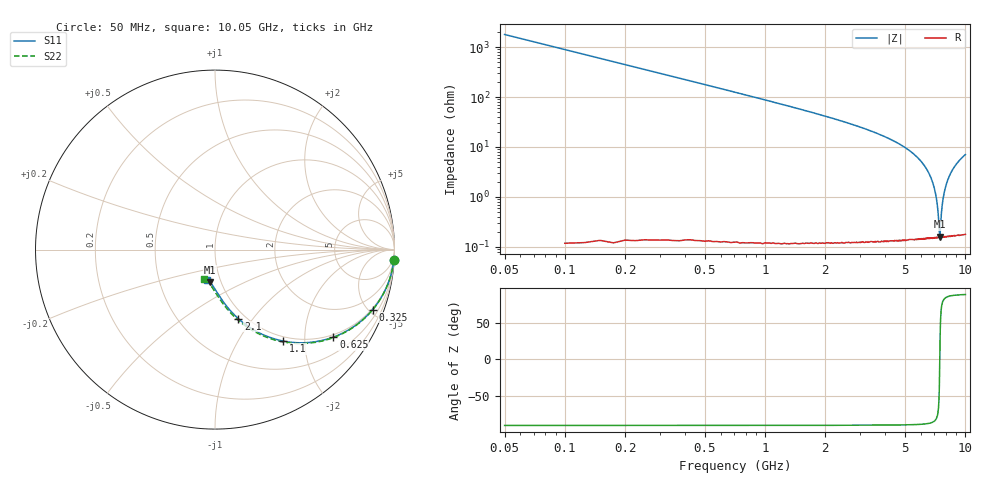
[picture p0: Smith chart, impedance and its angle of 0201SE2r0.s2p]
! AVX Thin Film Operation		Date: August 2001
! Description: Accu-P® Series, Thin Film, SMD, RF Capacitor
! Part Number: 02013J2R0ABW
! 50 MHz  -  10.05 GHz
! Serial Measurements
# mhz S db R 50
!	S11		S21		S12		S22
!	dB	Phase	dB	Phase	dB	Phase	dB	Phase
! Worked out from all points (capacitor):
!   401 points, 50 MHz to 10.05 GHz, reference 50 ohm
!   read as one part in series: C = 1.78 pF near 100 MHz
!   lowest |Z| = 160 mohm at 7.475 GHz (marker M1)
!   series resonance near 7.484 GHz, so ESL is about 250 pH
!   S11 on the Smith chart (normalised r, x): 50 MHz: 1, -34; 325 MHz: 0.93, -5.29; 625 MHz: 0.93, -2.76; 1.1 GHz: 0.93, -1.58; 2.1 GHz: 0.92, -0.85; 10.05 GHz: 0.86, -0.30
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50  -0.01 -3.3  -25.05 86.7  -25.05 86.7  -0.01 -3.4
75  -0.03 -5.0  -21.55 85.0  -21.55 85.0  -0.03 -5.0
125  -0.09 -8.3  -17.16 81.7  -17.16 81.7  -0.09 -8.4
150  -0.12 -9.9  -15.62 80.0  -15.62 80.0  -0.12 -10.0
175  -0.16 -11.5  -14.32 78.4  -14.32 78.4  -0.16 -11.6
250  -0.33 -16.3  -11.39 73.6  -11.39 73.6  -0.33 -16.4
325  -0.54 -20.8  -9.33 69.1  -9.33 69.1  -0.54 -21.0
450  -0.98 -27.9  -6.95 62.0  -6.95 62.0  -0.98 -28.1
625  -1.72 -36.5  -4.86 53.3  -4.86 53.3  -1.72 -36.8
825  -2.66 -44.6  -3.41 45.1  -3.41 45.1  -2.66 -45.1
1100  -3.95 -53.4  -2.25 36.2  -2.25 36.2  -3.95 -54.0
1400  -5.27 -60.5  -1.54 29.0  -1.54 29.0  -5.27 -61.3
1725  -6.55 -66.3  -1.10 23.1  -1.10 23.1  -6.55 -67.2
2100  -7.83 -71.3  -0.80 18.0  -0.80 18.0  -7.83 -72.5
2650  -9.38 -76.8  -0.55 12.3  -0.55 12.3  -9.38 -78.3
3400  -10.99 -82.2  -0.37 6.7  -0.37 6.7  -11.00 -84.0
4175  -12.22 -86.3  -0.28 2.3  -0.28 2.3  -12.23 -88.6
5050  -13.22 -90.1  -0.22 -1.8  -0.22 -1.8  -13.23 -92.8
6725  -14.37 -95.9  -0.17 -8.1  -0.17 -8.1  -14.39 -99.5
7475  -14.66 -98.2  -0.17 -10.6  -0.17 -10.6  -14.68 -102.1
8400  -14.88 -100.9  -0.16 -13.6  -0.16 -13.6  -14.90 -105.2
10050  -15.03 -105.3  -0.15 -18.4  -0.15 -18.4  -15.06 -110.3
